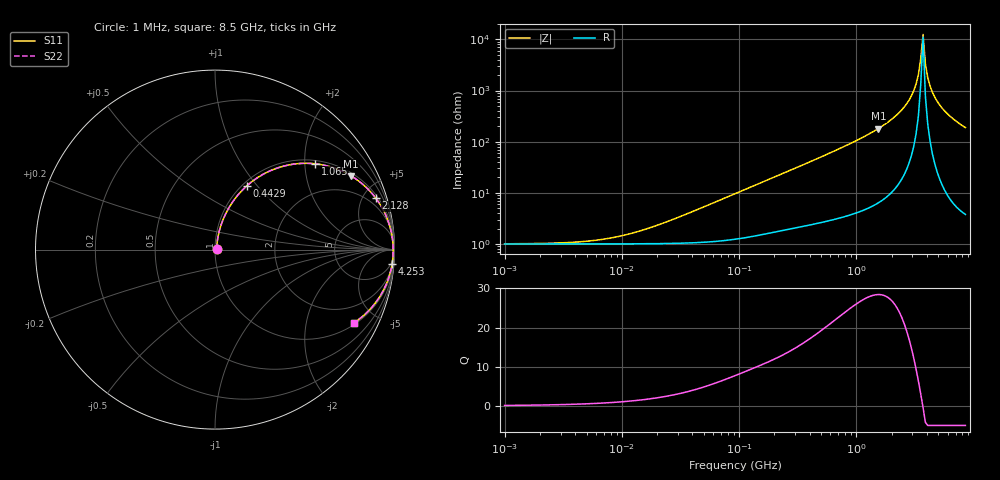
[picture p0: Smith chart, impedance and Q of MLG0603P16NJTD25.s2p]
! S-Parameter Data Generated by TDK Corporation
! Copyright(C) 2025 TDK Corporation.
! All Rights Reserved.
! TDK P/N: MLG0603P16NJTD25 (SMD / SMT Inductor (Coil))
! Property: L=16nH at 500MHz
! Size(LxWxT): 0.6x0.3x0.3mm
! Model Type: s2p (Touchstone File Format Version 1.0)
! Frequency: DC=Yes Start=1MHz Stop=8500MHz 198points Log-sweep
! Model Generated on Feb. 6, 2025
! Terms and conditions regarding TDK Simulation Models:
! 1)This simulation model is being provided solely for informational
!  purposes. Please refer to the specifications of the products in
!  terms of detailed characteristics of such products.
! 2)In no event shall TDK Corporation of any of its subsidiaries be
!  liable for any loss or damage arising, directly or indirectly,
!  from any information contained in this simulation model, including,
!  but not limited to loss or damages arising from any inaccuracies,
!  omissions or errors in connection with such information.
! 3)Any and all copyrights on this simulation model are owned by
!  TDK Corporation.  Duplication or redistribution of this simulation
!  model without prior written permission from TDK Corporation
!  is prohibited.
! 4)This simulation model is subject to any modification or change
!  without any prior notice.
! 5)Neither TDK Corporation nor any of its subsidiaries shall make any
!  warranty, express or implied, including but not limited to the
!  correctness, implied warranties of merchantability and fitness for
!  a particular purpose with respect to this simulation models.
! 6)The use of this simulation model shall be deemed to have consented
!  to the terms and conditions hereof.
! Port Assignments:
!  1 ---@@@--- 2
! Applicable Conditions:
!  Temperature = 25 degC
!  DC Bias Current = 0 A
!  Small Signal Operation
# Hz S MA R 50
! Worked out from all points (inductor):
!   197 points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, 1 MHz to 8.5 GHz, reference 50 ohm
!   read as one part in series: L = 16.6 nH near 30.45 MHz
!   highest Q = 28.4 at 1.54 GHz (marker M1), where L = 18.7 nH
!   self-resonance near 3.536 GHz
!   S11 on the Smith chart (normalised r, x): 1 MHz: 1.02, +0.00; 442.9 MHz: 1.05, +0.89; 1.065 GHz: 1.09, +2.26; 2.128 GHz: 1.24, +6.18; 4.253 GHz: 3, -24; 8.5 GHz: 1.08, -3.77
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1000000  0.009955 5.9  0.9901 -0.1  0.9901 -0.1  0.009955 5.9
4587603  0.01098 25.3  0.9901 -0.3  0.9901 -0.3  0.01098 25.3
9601846  0.01403 44.4  0.99 -0.6  0.99 -0.6  0.01403 44.4
2.10461e7  0.02391 63.9  0.9897 -1.2  0.9897 -1.2  0.02391 63.9
9.219544e7  0.09436 77.2  0.9835 -5.4  0.9835 -5.4  0.09436 77.2
4.229561e8  0.3835 64.2  0.9021 -22.5  0.9021 -22.5  0.3835 64.2
4.429384e8  0.3987 63.4  0.8953 -23.5  0.8953 -23.5  0.3987 63.4
1.064771e9  0.736 40.5  0.6499 -47.3  0.6499 -47.3  0.736 40.5
1.540426e9  0.8627 28.4  0.4762 -59.6  0.4762 -59.6  0.8627 28.4
1.940355e9  0.9221 20.8  0.3546 -67.1  0.3546 -67.1  0.9221 20.8
2.128028e9  0.9408 17.7  0.3044 -70.1  0.3044 -70.1  0.9408 17.7
2.80715e9  0.9797 8.7  0.1514 -78.0  0.1514 -78.0  0.9797 8.7
3.224109e9  0.9894 4.2  0.07437 -79.7  0.07437 -79.7  0.9894 4.2
3.37643e9  0.9913 2.8  0.04876 -78.3  0.04876 -78.3  0.9913 2.8
3.535948e9  0.9924 1.3  0.02352 -70.6  0.02352 -70.6  0.9924 1.3
3.703002e9  0.9929 -0.2  0.007927 25.9  0.007927 25.9  0.9929 -0.2
3.877948e9  0.9926 -1.7  0.03016 75.0  0.03016 75.0  0.9926 -1.7
4.061159e9  0.9917 -3.2  0.05565 79.8  0.05565 79.8  0.9917 -3.2
4.253027e9  0.99 -4.7  0.0814 80.6  0.0814 80.6  0.99 -4.7
4.664383e9  0.9845 -7.6  0.1331 79.5  0.1331 79.5  0.9845 -7.6
5.357206e9  0.9709 -12.2  0.2109 76.0  0.2109 76.0  0.9709 -12.2
8.5e9  0.8761 -27.7  0.4649 61.1  0.4649 61.1  0.8761 -27.7
